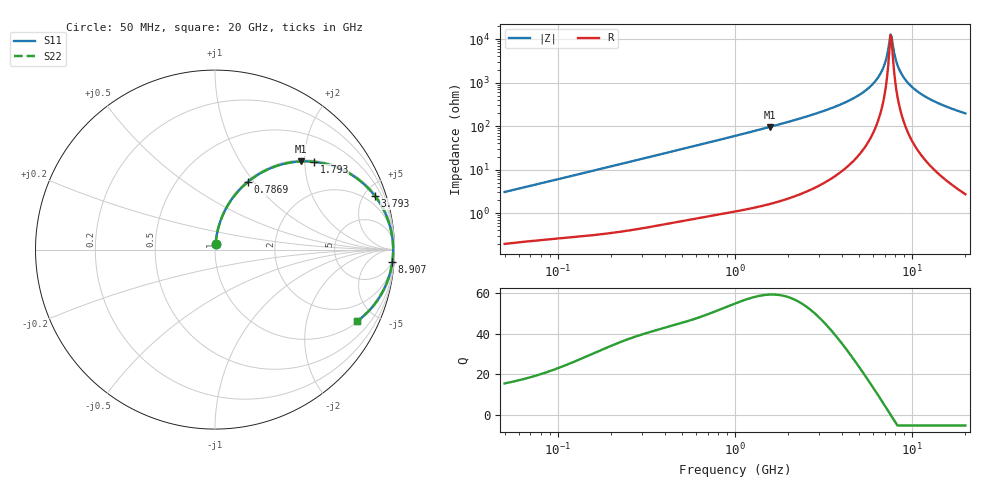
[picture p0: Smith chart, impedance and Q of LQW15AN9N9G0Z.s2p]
!Murata Part Number: LQW15AN9N9G0Z
!These Parameters are Measured in Series Mode Connection
!  o--[Z]--o
!Port1  Port2
!  o-------o
!Freq. Start=50[MHz] Stop=20[GHz], 401[Steps]
# Hz S RI R 50
!Freq.(Hz) S11(Real) S11(Imag) S21(Real) S21(Imag) S12(Real) S12(Imag) S22(Real) S22(Imag)
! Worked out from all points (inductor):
!   401 points, 50 MHz to 20 GHz, reference 50 ohm
!   read as one part in series: L = 9.67 nH near 51.52 MHz
!   highest Q = 59.2 at 1.567 GHz (marker M1), where L = 9.71 nH
!   self-resonance near 7.554 GHz
!   S11 on the Smith chart (normalised r, x): 50 MHz: 1.00, +0.06; 786.9 MHz: 1.02, +0.93; 1.793 GHz: 1.04, +2.22; 3.793 GHz: 1.16, +5.89; 8.907 GHz: 4, -27; 20 GHz: 1.05, -3.92
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5e7  0.00289 0.0304  0.9971 -0.0304  0.9971 -0.0304  0.00289 0.0304
1.364002e8  0.00949 0.0806  0.9905 -0.0806  0.9905 -0.0806  0.00949 0.0806
3.721004e8  0.051 0.2085  0.949 -0.2085  0.949 -0.2085  0.051 0.2085
7.868965e8  0.1837 0.3776  0.8163 -0.3776  0.8163 -0.3776  0.1837 0.3776
1e9  0.2659 0.4328  0.7341 -0.4328  0.7341 -0.4328  0.2659 0.4328
1.567309e9  0.478 0.4911  0.522 -0.4911  0.522 -0.4911  0.478 0.4911
1.793498e9  0.5506 0.489  0.4494 -0.489  0.4494 -0.489  0.5506 0.489
2.728004e9  0.765 0.4143  0.235 -0.4143  0.235 -0.4143  0.765 0.4143
3.792786e9  0.8904 0.2995  0.1096 -0.2995  0.1096 -0.2995  0.8904 0.2995
5.041459e9  0.9579 0.1807  0.0421 -0.1807  0.0421 -0.1807  0.9579 0.1807
6.125241e9  0.9831 0.0953  0.0169 -0.0953  0.0169 -0.0953  0.9831 0.0953
6.601595e9  0.9885 0.0621  0.0115 -0.0621  0.0115 -0.0621  0.9885 0.0621
6.905011e9  0.9907 0.0422  0.00933 -0.0422  0.00933 -0.0422  0.9907 0.0422
7.114996e9  0.9917 0.0288  0.00834 -0.0288  0.00834 -0.0288  0.9917 0.0288
7.442007e9  0.9925 0.00883  0.00753 -0.00883  0.00753 -0.00883  0.9925 0.00883
7.668323e9  0.9926 -0.00452  0.00744 0.00452  0.00744 0.00452  0.9926 -0.00452
8.264682e9  0.9912 -0.0379  0.0088 0.0379  0.0088 0.0379  0.9912 -0.0379
8.907419e9  0.9876 -0.0712  0.0124 0.0712  0.0124 0.0712  0.9876 -0.0712
1.004137e10  0.977 -0.1243  0.023 0.1243  0.023 0.1243  0.977 -0.1243
1.183995e10  0.9524 -0.1964  0.0476 0.1964  0.0476 0.1964  0.9524 -0.1964
1.504638e10  0.8945 -0.2967  0.1055 0.2967  0.1055 0.2967  0.8945 -0.2967
2e10  0.7904 -0.4001  0.2096 0.4001  0.2096 0.4001  0.7904 -0.4001
